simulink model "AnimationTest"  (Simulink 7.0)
settings: Solver=FixedStepDiscrete  StartTime=0.0  StopTime=inf  FixedStep=samplePeriod  RelTol=1e-3
PreLoadFcn:
  | initialize
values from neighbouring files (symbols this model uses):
  samplePeriod = controlPeriod/upsampleFactor    (= 0.00048828125)    [initialize.m]    (also in viewer.m = eval(getHeaderValue(header, 'DELTA_T')))
  x = []    [loadbin.m]    (also in player.m = xPanel + panelWide + margin; quake.m = 365; resondemo.m = xOrigin + marginWide + panelWide + plotMarginWide; sinefit.m = 2 * pi * freq * (0:npoints-1)' * deltaT)
  yaw = drot(3) * canon    [animation.m]    (also in eulerRot.m)
undefined symbols (not defined in the file or in its folder): animation, DiscIntNeverNeededParam

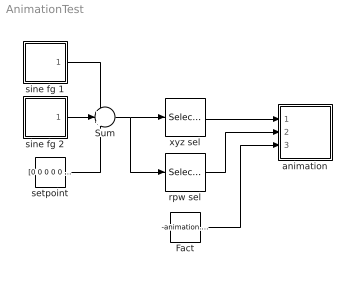
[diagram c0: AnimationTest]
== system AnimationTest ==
  Fact : Constant  Value=-animation.fmax  OutDataType=sfix(16)  OutScaling=2^0
  Sum : Sum  Inputs=+++  OutDataType=sfix(16)  OutScaling=2^0
  animation : Subsystem  mask{azim=-37.5, elev=35, params=animation, decim=ceil((1/samplePeriod)/32), samplePeriod=samplePeriod}
      mask prompts: azim "View azimuth (degrees)"; elev "View elevation (degrees)"; params "Parameters"; decim "Decimation factor"; samplePeriod "Sample period (sec)"
  rpw sel : Selector  InputPortWidth=6  IndexOptions=Index vector (dialog)  Indices=[4 5 6]  OutputSizes=1
  setpoint : Constant  Value=[0 0 0 0 0 0]  OutDataType=sfix(16)  OutScaling=2^0
  sine fg 1 : Subsystem  mask(Sine Function Generator){id=yaw, ampl=15, freq=0.25, phase=0, spanInterval=1, samplePeriod=samplePeriod}
      mask prompts: id "DOF"; ampl "Amplitude"; freq "Frequency (Hz)"; phase "Phase (deg)"; spanInterval "Span interval (sec)"; samplePeriod "Sample period (sec)"
  sine fg 2 : Subsystem  mask(Sine Function Generator){id=x, ampl=0, freq=0.25, phase=0, spanInterval=1, samplePeriod=samplePeriod}
      mask prompts: id "DOF"; ampl "Amplitude"; freq "Frequency (Hz)"; phase "Phase (deg)"; spanInterval "Span interval (sec)"; samplePeriod "Sample period (sec)"
  xyz sel : Selector  InputPortWidth=6  IndexOptions=Index vector (dialog)  Indices=[1 2 3]  OutputSizes=1
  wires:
  Fact/1 -> animation/3(Fact)
  setpoint/1 -> Sum/3
  sine fg 1/1(out) -> Sum/1
  sine fg 2/1(out) -> Sum/2
  Sum/1 -> xyz sel/1, rpw sel/1
  xyz sel/1 -> animation/1(xyz)
  rpw sel/1 -> animation/2(rpw)

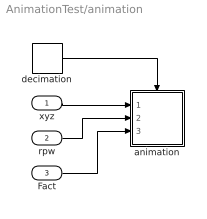
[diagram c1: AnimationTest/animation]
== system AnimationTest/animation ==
  xyz : Inport
  rpw : Inport  Port=2
  Fact : Inport  Port=3
  animation : Subsystem  TreatAsAtomicUnit=on
  decimation : DiscretePulseGenerator  Period=decim  SampleTime=samplePeriod
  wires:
  decimation/1 -> animation/Trigger
  xyz/1 -> animation/1(xyz)
  Fact/1 -> animation/3(Fact)
  rpw/1 -> animation/2(rpw)

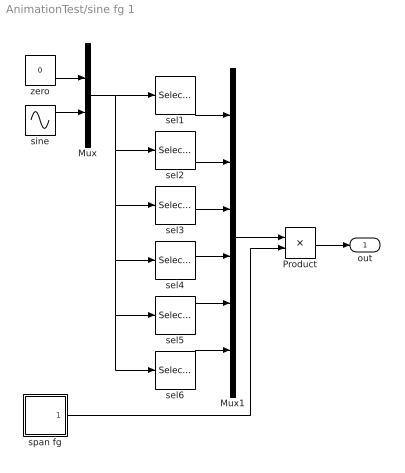
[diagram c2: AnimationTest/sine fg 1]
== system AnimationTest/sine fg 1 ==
  Mux : Mux  Inputs=2
  Mux1 : Mux  Inputs=6
  Product : Product  OutDataType=sfix(16)  OutScaling=2^0
  sel1 : Selector  InputPortWidth=2  IndexOptions=Index vector (dialog)  Indices=(id==1)+1  OutputSizes=1
  sel2 : Selector  InputPortWidth=2  IndexOptions=Index vector (dialog)  Indices=(id==2)+1  OutputSizes=1
  sel3 : Selector  InputPortWidth=2  IndexOptions=Index vector (dialog)  Indices=(id==3)+1  OutputSizes=1
  sel4 : Selector  InputPortWidth=2  IndexOptions=Index vector (dialog)  Indices=(id==4)+1  OutputSizes=1
  sel5 : Selector  InputPortWidth=2  IndexOptions=Index vector (dialog)  Indices=(id==5)+1  OutputSizes=1
  sel6 : Selector  InputPortWidth=2  IndexOptions=Index vector (dialog)  Indices=(id==6)+1  OutputSizes=1
  sine : Sin  Amplitude=ampl  Frequency=2 * pi * freq  Phase=phase*180/pi  SampleTime=samplePeriod
  span fg : Subsystem  mask{spanInterval=spanInterval, samplePeriod=samplePeriod}
      mask prompts: spanInterval "Span interval (sec)"; samplePeriod "Sample period (sec)"
  zero : Constant  Value=0  OutDataType=sfix(16)  OutScaling=2^0  SampleTime=samplePeriod
  out : Outport  OutDataType=sfix(16)  OutScaling=2^0
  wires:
  span fg/1(out) -> Product/2
  Product/1 -> out/1
  Mux1/1 -> Product/1
  zero/1 -> Mux/1
  sine/1 -> Mux/2
  sel1/1 -> Mux1/1
  sel2/1 -> Mux1/2
  sel3/1 -> Mux1/3
  sel4/1 -> Mux1/4
  sel5/1 -> Mux1/5
  sel6/1 -> Mux1/6
  Mux/1 -> sel2/1, sel3/1, sel4/1, sel5/1, sel6/1, sel1/1

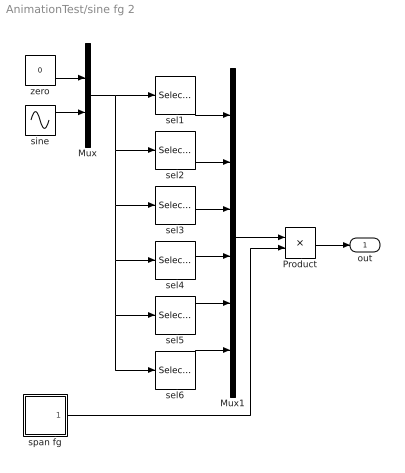
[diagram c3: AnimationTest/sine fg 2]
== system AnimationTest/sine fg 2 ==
  Mux : Mux  Inputs=2
  Mux1 : Mux  Inputs=6
  Product : Product  OutDataType=sfix(16)  OutScaling=2^0
  sel1 : Selector  InputPortWidth=2  IndexOptions=Index vector (dialog)  Indices=(id==1)+1  OutputSizes=1
  sel2 : Selector  InputPortWidth=2  IndexOptions=Index vector (dialog)  Indices=(id==2)+1  OutputSizes=1
  sel3 : Selector  InputPortWidth=2  IndexOptions=Index vector (dialog)  Indices=(id==3)+1  OutputSizes=1
  sel4 : Selector  InputPortWidth=2  IndexOptions=Index vector (dialog)  Indices=(id==4)+1  OutputSizes=1
  sel5 : Selector  InputPortWidth=2  IndexOptions=Index vector (dialog)  Indices=(id==5)+1  OutputSizes=1
  sel6 : Selector  InputPortWidth=2  IndexOptions=Index vector (dialog)  Indices=(id==6)+1  OutputSizes=1
  sine : Sin  Amplitude=ampl  Frequency=2 * pi * freq  Phase=phase*180/pi  SampleTime=samplePeriod
  span fg : Subsystem  mask{spanInterval=spanInterval, samplePeriod=samplePeriod}
      mask prompts: spanInterval "Span interval (sec)"; samplePeriod "Sample period (sec)"
  zero : Constant  Value=0  OutDataType=sfix(16)  OutScaling=2^0  SampleTime=samplePeriod
  out : Outport  OutDataType=sfix(16)  OutScaling=2^0
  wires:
  Mux/1 -> sel1/1, sel6/1, sel5/1, sel4/1, sel3/1, sel2/1
  sel6/1 -> Mux1/6
  sel5/1 -> Mux1/5
  sel4/1 -> Mux1/4
  sel3/1 -> Mux1/3
  sel2/1 -> Mux1/2
  sel1/1 -> Mux1/1
  sine/1 -> Mux/2
  zero/1 -> Mux/1
  Mux1/1 -> Product/1
  Product/1 -> out/1
  span fg/1(out) -> Product/2

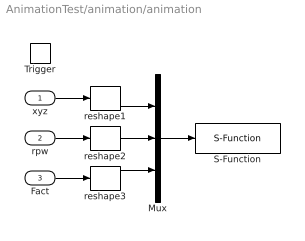
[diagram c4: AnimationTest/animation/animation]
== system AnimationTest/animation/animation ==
  xyz : Inport  OutDataType=sfix(16)  OutScaling=2^0
  rpw : Inport  Port=2  OutDataType=sfix(16)  OutScaling=2^0
  Fact : Inport  Port=3  OutDataType=sfix(16)  OutScaling=2^0
  Trigger : TriggerPort
  Mux : Mux  Inputs=3
  S-Function : S-Function  FunctionName=animation  Parameters=azim,elev,params
  reshape1 : Reshape
  reshape2 : Reshape
  reshape3 : Reshape
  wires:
  Mux/1 -> S-Function/1
  xyz/1 -> reshape1/1
  Fact/1 -> reshape3/1
  reshape3/1 -> Mux/3
  rpw/1 -> reshape2/1
  reshape2/1 -> Mux/2
  reshape1/1 -> Mux/1

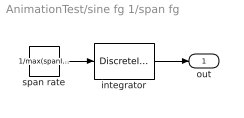
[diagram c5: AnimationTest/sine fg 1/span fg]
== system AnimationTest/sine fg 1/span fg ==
  integrator : DiscreteIntegrator  SampleTime=samplePeriod  OutDataType=sfix(16)  OutScaling=2^0  LimitOutput=on  UpperSaturationLimit=1  LowerSaturationLimit=0  ICPrevOutput=DiscIntNeverNeededParam  ICPrevScaledInput=DiscIntNeverNeededParam
  span rate : Constant  Value=1/max(spanInterval,samplePeriod)  OutDataType=sfix(16)  OutScaling=2^0  SampleTime=samplePeriod
  out : Outport  OutDataType=sfix(16)  OutScaling=2^0
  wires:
  span rate/1 -> integrator/1
  integrator/1 -> out/1

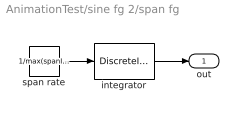
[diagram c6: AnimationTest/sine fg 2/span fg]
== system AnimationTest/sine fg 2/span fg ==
  integrator : DiscreteIntegrator  SampleTime=samplePeriod  OutDataType=sfix(16)  OutScaling=2^0  LimitOutput=on  UpperSaturationLimit=1  LowerSaturationLimit=0  ICPrevOutput=DiscIntNeverNeededParam  ICPrevScaledInput=DiscIntNeverNeededParam
  span rate : Constant  Value=1/max(spanInterval,samplePeriod)  OutDataType=sfix(16)  OutScaling=2^0  SampleTime=samplePeriod
  out : Outport  OutDataType=sfix(16)  OutScaling=2^0
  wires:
  integrator/1 -> out/1
  span rate/1 -> integrator/1
